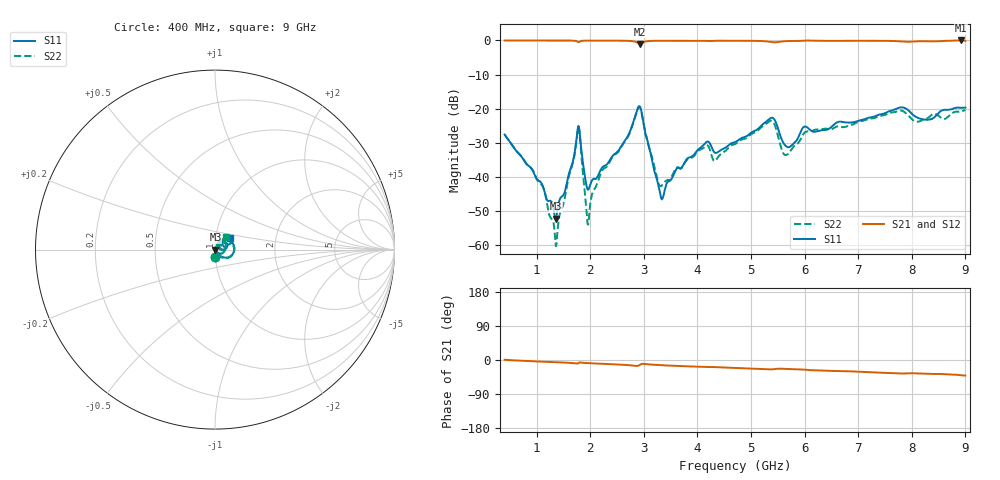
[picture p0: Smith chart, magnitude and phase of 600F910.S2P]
!  American Technical Ceramics  Date:  11/7/05
!  One Norden Lane
!  Huntington Station,  NY.  11746-2102
!  Tel:  (631) 622-4700  Fax:  (631) 622-4748
!  Part Number  600F910  Mounting Orientation: Horizontal
!  Description: Ultra Low ESR Microwave capacitors
!  Application: Coupling, Bypass, Tuning, DC Block
!  Filters, Matching
# GHZ S DB R 50
! Freq  |S11|  S11 Ph  |S21|  S21 Ph  |S12|  S12 Ph  |S22|  S22 Ph
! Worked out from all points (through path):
!   801 points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, 400 MHz to 9 GHz, reference 50 ohm
!   highest |S21| = 0.00 dB at 8.914 GHz (marker M1); lowest = -1.0 dB at 2.926 GHz (marker M2)
!   group delay of S21, straight-line fit = 12.5 ps
!   lowest |S11| = -52.3 dB at 1.357 GHz (marker M3), VSWR 1.00, Z = 50.2 - j0.0139 ohm
!   |S11| at or under -10 dB: start of sweep to end of sweep
!   |S22| runs from -60.3 to -19.4 dB; largest |S21 - S12| = 0.008
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0.4  -27.59 -88.4  -0.01 0.7  -0.02 0.7  -27.56 -88.7
1.11  -42.59 -79.0  -0.01 -4.4  -0.02 -4.5  -42.76 -93.0
1.357  -52.27 -3.2  -0.02 -5.8  -0.02 -5.9  -60.34 -21.0
1.54  -43.38 52.9  -0.03 -6.9  -0.03 -7.0  -44.74 67.5
1.755  -27.19 39.5  -0.27 -9.3  -0.27 -9.3  -27.64 35.8
1.841  -33.23 -47.2  -0.12 -6.9  -0.12 -7.0  -35.27 -66.8
1.927  -42.47 -26.2  -0.05 -8.0  -0.05 -8.1  -49.59 -65.2
1.97  -43.58 5.6  -0.04 -8.4  -0.05 -8.5  -52.65 24.6
2.206  -37.60 47.7  -0.05 -9.9  -0.05 -10.0  -38.58 70.1
2.926  -19.43 -6.0  -1.00 -12.5  -1.00 -12.7  -19.59 -10.1
3.27  -42.57 -41.0  -0.08 -13.3  -0.08 -13.5  -41.82 -38.1
3.346  -46.40 5.5  -0.07 -13.9  -0.07 -14.1  -42.27 -7.5
4.163  -29.84 50.4  -0.14 -18.6  -0.14 -18.9  -30.83 39.6
4.324  -32.91 39.9  -0.11 -18.7  -0.11 -18.9  -35.34 42.1
4.7  -29.81 57.1  -0.07 -20.9  -0.08 -21.2  -30.43 64.2
5.377  -22.68 28.1  -0.45 -24.9  -0.45 -25.1  -23.52 27.5
5.657  -31.06 20.4  -0.20 -23.6  -0.21 -23.9  -33.58 38.9
6.141  -26.65 39.0  -0.06 -27.0  -0.06 -27.3  -26.52 58.3
7.57  -20.81 43.9  -0.13 -34.5  -0.14 -34.9  -21.39 51.2
8.291  -23.25 35.9  -0.23 -36.6  -0.23 -37.0  -22.82 49.0
8.914  -19.75 38.7  0.00 -40.2  0.00 -40.6  -20.87 48.4
9  -19.69 37.9  -0.11 -40.9  -0.11 -41.4  -20.38 48.3
